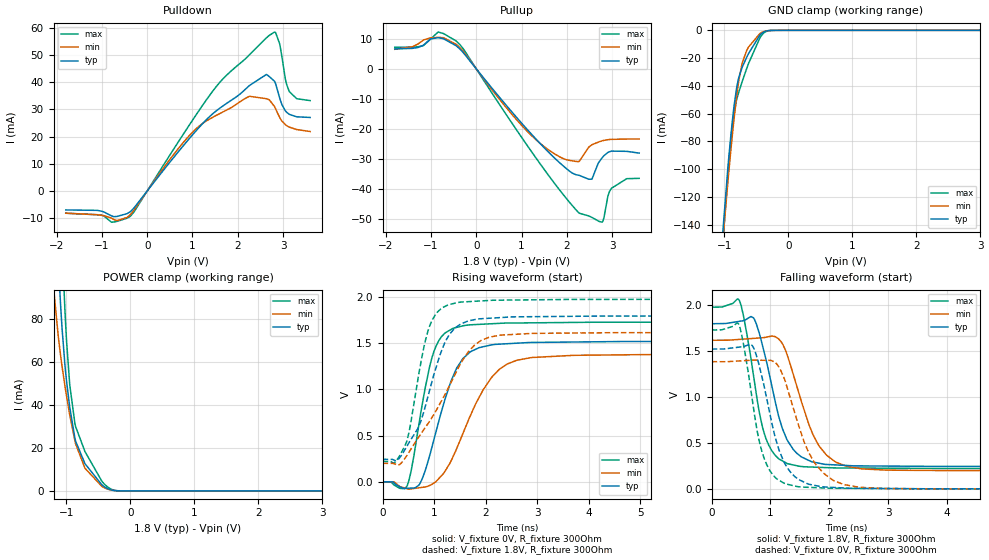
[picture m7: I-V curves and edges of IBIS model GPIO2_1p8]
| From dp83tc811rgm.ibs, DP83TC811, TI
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|   GPIO2_1p8 Model
[Model]   GPIO2_1p8
Model_type   I/O
Polarity   Non-Inverting
Enable   Active-Low
Vinl = 0.63
Vinh = 1.17
Vmeas = 0.9
Vref = 0
Cref = 2pF
Rref = 100000
|   typ   min   max
C_comp   3.2934pF   3.1163pF   3.4328pF
[Model spec]
|subparameter
Vinl   0.63   0.567   0.693
Vinh   1.17   1.053   1.287
| Where Nom  PVT is Nominal Process, 1.8V, 27C
|   Fast PVT is Strong Process,  1.98V, -40C
|   Slow PVT is Weak Process,   1.62V, 125C
[Voltage Range]   1.8   1.62   1.98
|Junction Temperature
[Temperature Range]   27   125   -40
[Pullup Reference]   1.8   1.62   1.98
[Pulldown Reference]   0   0   0
[Power Clamp Reference]   1.8   1.62   1.98
[GND Clamp Reference]   0   0   0
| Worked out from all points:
|   slope of the pulldown table from 0 to 0.27 V, typ, clamps not added: 46.9 ohm
|   slope of the pullup table from 0 to 0.27 V, typ, clamps not added: 53.6 ohm
|   GND clamp passes 1 mA (typ) near -0.38 V on its own axis
|   POWER clamp passes 1 mA (typ) near -0.35 V on its own axis
|   falling waveform, V_fixture 1.8V, R_fixture 300Ohm: 20-80 % time 376ps typ, 467ps min, 297ps max; typ from 1.8 V to 0.243 V
|   rising waveform, V_fixture 0V, R_fixture 300Ohm: 20-80 % time 504ps typ, 717ps min, 355ps max; typ from 0 V to 1.52 V
|   rising waveform, V_fixture 1.8V, R_fixture 300Ohm: 20-80 % time 533ps typ, 876ps min, 353ps max; typ from 0.243 V to 1.8 V
|   falling waveform, V_fixture 0V, R_fixture 300Ohm: 20-80 % time 367ps typ, 479ps min, 294ps max; typ from 1.52 V to 0 V
[Pulldown]
|   Voltage   I(typ)   I(min)   I(max)
-1.8V     -7.008mA   -8.193mA   -8.22mA
-790.2mV  -9.174mA   -9.982mA   -11.52mA
-369mV    -7.582mA   -8.668mA   -9.241mA
689.4mV   14.47mA    15.65mA    18.12mA
1.219V    24.7mA     24.79mA    31.42mA
2.261V    38.86mA    34.85mA    50.19mA
2.633V    42.9mA     33.96mA    56.38mA
2.812V    40.39mA    31.1mA     58.51mA
2.925V    34.3mA     27.07mA    54.23mA
3.049V    29.56mA    24.45mA    41.43mA
3.141V    28.2mA     23.49mA    36.55mA
3.6V      27.06mA    21.89mA    33.27mA
[GND Clamp]
|   Voltage   I(typ)   I(min)   I(max)
-1.8V     -712.6mA   -651.3mA   -757.4mA
-1.055V   -163.2mA   -167.9mA   -171.7mA
-941.4mV  -96.91mA   -107.3mA   -101.5mA
-898.2mV  -75.54mA   -86.1mA    -78.92mA
-865.8mV  -61.29mA   -71.17mA   -65.16mA
-811.8mV  -42.38mA   -48.94mA   -50.64mA
-779.4mV  -34.85mA   -37.85mA   -45.22mA
-720mV    -26.4mA    -23.4mA    -36.68mA
-649.8mV  -19.25mA   -14.35mA   -27.31mA
-423mV    -2.44mA    -1.697mA   -3.918mA
-228.6mV  -30.06uA   -39.9uA    -34.02uA
3.6V      0A         0A         0A
[Pullup]
|   Voltage   I(typ)   I(min)   I(max)
-1.8V     6.631mA    6.523mA    7.204mA
-1.168V   7.883mA    9.608mA    7.743mA
-844.2mV  10.4mA     10.5mA     12.25mA
-444.6mV  7.711mA    8.202mA    9.312mA
1.246V    -22.25mA   -22.63mA   -28.18mA
1.84V     -31.33mA   -29.35mA   -40.42mA
2.277V    -35.59mA   -30.89mA   -48.22mA
2.552V    -36.85mA   -25.39mA   -49.6mA
2.779V    -29.76mA   -24.06mA   -51.22mA
2.909V    -27.93mA   -23.67mA   -42.47mA
2.984V    -27.5mA    -23.56mA   -39.97mA
3.6V      -28.15mA   -23.44mA   -36.57mA
[POWER Clamp]
|   Voltage   I(typ)   I(min)   I(max)
-1.8V     697.7mA    523.7mA    835.7mA
-1.19V    150.3mA    91.9mA     220.1mA
-1.093V   88.3mA     63.89mA    135.3mA
-1.066V   75.39mA    57.89mA    114.3mA
-1.022V   58.97mA    49.12mA    84.66mA
-995.4mV  50.88mA    44.02mA    69.49mA
-946.8mV  39.06mA    35.47mA    49.51mA
-860.4mV  23.92mA    22.65mA    30.7mA
-709.2mV  12.71mA    10.59mA    18.39mA
-417.6mV  2.205mA    1.66mA     3.564mA
-169.2mV  37.16uA    43.49uA    57.95uA
3.6V      0A         0A         0A
[Ramp]
R_load = 300
|   typ   min   max
dV/dt_r   0.914244/5.02485e-10   0.831302/7.14301e-10   1.03881/3.53689e-10
dV/dt_f   0.933424/3.73944e-10   0.851745/4.66369e-10   1.05488/2.96294e-10
[Falling Waveform]
V_fixture = 1.8V
V_fixture_min = 1.62V
V_fixture_max = 1.98V
R_fixture = 300Ohm
C_fixture = 0F
|   Time   V(typ)   V(min)   V(max)
0s        1.799V     1.619V     1.979V
470.4ps   1.825V     1.629V     2.054V
719.5ps   1.857V     1.64V      1.209V
861.9ps   1.572V     1.647V     685mV
970.2ps   1.284V     1.658V     480.6mV
1.202ns   663.1mV    1.584V     308.7mV
1.488ns   370.8mV    1.038V     249.5mV
1.956ns   268.8mV    369.2mV    234.4mV
2.573ns   252.9mV    219.9mV    229.6mV
20ns      243.3mV    199.8mV    220.9mV
[Rising Waveform]
V_fixture = 0V
V_fixture_min = 0V
V_fixture_max = 0V
R_fixture = 300Ohm
C_fixture = 0F
|   Time   V(typ)   V(min)   V(max)
0s        108.1uV    278.6uV    49.23uV
470.4ps   -70.93mV   -73.94mV   -51.47mV
712.4ps   -31.49mV   -65.25mV   642.9mV
917.4ps   288.6mV    -39.48mV   1.255V
1.045ns   557.3mV    6.185mV    1.478V
1.334ns   1.096V     229.7mV    1.651V
1.573ns   1.341V     539.7mV    1.691V
2.135ns   1.484V     1.141V     1.712V
2.904ns   1.509V     1.346V     1.721V
20ns      1.524V     1.386V     1.731V
[Rising Waveform]
V_fixture = 1.8V
V_fixture_min = 1.62V
V_fixture_max = 1.98V
R_fixture = 300Ohm
C_fixture = 0F
|   Time   V(typ)   V(min)   V(max)
0s        243.3mV    199.8mV    220.9mV
234.7ps   232.1mV    193.8mV    207.7mV
460.1ps   372.5mV    273.1mV    422.5mV
795.6ps   747.2mV    560.4mV    1.438V
957.9ps   1.082V     694.6mV    1.746V
1.202ns   1.498V     934.8mV    1.896V
1.454ns   1.684V     1.215V     1.941V
1.919ns   1.766V     1.532V     1.959V
2.914ns   1.788V     1.607V     1.971V
20ns      1.799V     1.618V     1.979V
[Falling Waveform]
|Gnd
V_fixture = 0V
V_fixture_min = 0V
V_fixture_max = 0V
R_fixture = 300Ohm
C_fixture = 0F
|   Time   V(typ)   V(min)   V(max)
0s        1.524V     1.386V     1.732V
460.1ps   1.544V     1.394V     1.797V
697.1ps   1.557V     1.403V     951.5mV
800.9ps   1.367V     1.403V     551.1mV
941.4ps   973.9mV    1.401V     261.2mV
1.15ns    419.9mV    1.323V     96.11mV
1.454ns   117.3mV    744.3mV    28.37mV
1.9ns     24.81mV    174.9mV    13.17mV
2.529ns   8.837mV    19.99mV    8.223mV
20ns      108.9uV    297.4uV    49.83uV
